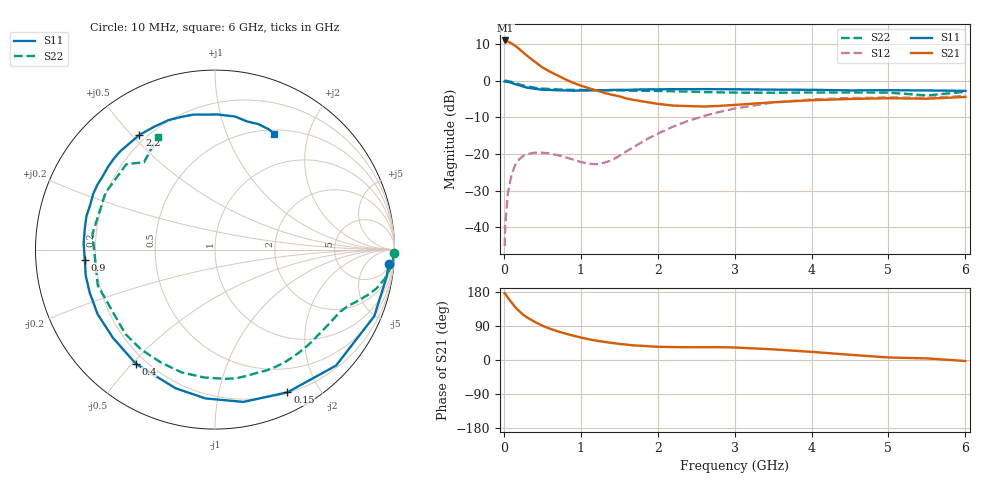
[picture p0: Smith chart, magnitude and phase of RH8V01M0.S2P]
! SIEMENS Small Signal Semiconductors
! BFR106
! Si NPN RF Bipolar Junction Transistor in SOT23
! VCE = 8 V  IC = 1 mA
! Common Emitter S-Parameters:  August  1996
# GHz  S  MA  R  50
!  f  S11  S21  S12  S22
! GHz  MAG  ANG  MAG  ANG  MAG  ANG  MAG  ANG
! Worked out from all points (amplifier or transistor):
!   36 points, 10 MHz to 6 GHz, reference 50 ohm
!   highest |S21| = 11.0 dB at 20 MHz (marker M1)
!   |S21| within 3 dB of that: start of sweep to 236.5 MHz
!   unconditionally stable (mu >= 1): 858.4 MHz to 1.864 GHz; 3.058 GHz to end of sweep
!   at 250 MHz: K = 0.26, MSG = 14.1 dB, |S12| = -20.6 dB
!   at 1.4 GHz: K = 1.40, MAG = 5.2 dB, |S12| = -21.7 dB
!   at 6 GHz: K = 1.02, MAG = -0.9 dB, |S12| = -4.2 dB
!   S11 on the Smith chart (normalised r, x): 10 MHz: 8, -22; 150 MHz: 0.21, -1.61; 400 MHz: 0.16, -0.51; 900 MHz: 0.16, -0.04; 2.2 GHz: 0.17, +0.53; 6 GHz: 0.55, +1.49
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0.01  0.9715 -4.6  3.499 176.4  0.0055 87.2  0.9999 -1.1
0.02  0.9683 -9.1  3.534 174.2  0.0111 84.9  0.9968 -2.1
0.05  0.9619 -22.7  3.426 164.9  0.028 77.5  0.9869 -5.2
0.1  0.934 -43.8  3.222 152.0  0.0522 66.1  0.9604 -9.7
0.15  0.8918 -63.1  2.974 138.8  0.0713 54.9  0.9248 -13.6
0.2  0.8632 -79.4  2.701 129.1  0.0845 47.3  0.8909 -16.3
0.25  0.8309 -93.7  2.432 119.7  0.0938 40.3  0.8602 -18.6
0.3  0.8031 -105.9  2.196 112.5  0.099 35.2  0.8366 -20.4
0.4  0.7739 -124.8  1.818 100.8  0.104 27.2  0.8005 -23.4
0.5  0.7514 -139.3  1.518 90.6  0.1038 22.2  0.7794 -26.3
0.6  0.7464 -151.2  1.324 82.5  0.1012 19.4  0.7677 -29.4
0.9  0.7275 -175.6  0.935 64.4  0.0837 21.9  0.7468 -39.2
1.1  0.7348 171.0  0.791 54.9  0.0736 33.6  0.7424 -46.7
1.3  0.7385 160.2  0.684 48.1  0.0754 53.3  0.7387 -54.5
1.6  0.7474 146.5  0.568 40.5  0.1091 75.1  0.7317 -66.9
2.2  0.7652 123.4  0.456 34.1  0.2355 77.7  0.7153 -94.7
2.8  0.7628 104.4  0.452 33.9  0.3735 63.7  0.6922 -126.5
3.5  0.753 89.0  0.506 28.1  0.5025 44.7  0.683 -163.1
4.5  0.7358 75.8  0.562 13.8  0.5788 20.6  0.6872 152.6
5  0.74 71.0  0.575 6.7  0.5898 11.5  0.6857 136.1
5.5  0.7342 66.0  0.566 4.2  0.5844 7.2  0.6271 129.1
6  0.725 62.9  0.599 -2.7  0.6159 -1.0  0.7043 117.0
